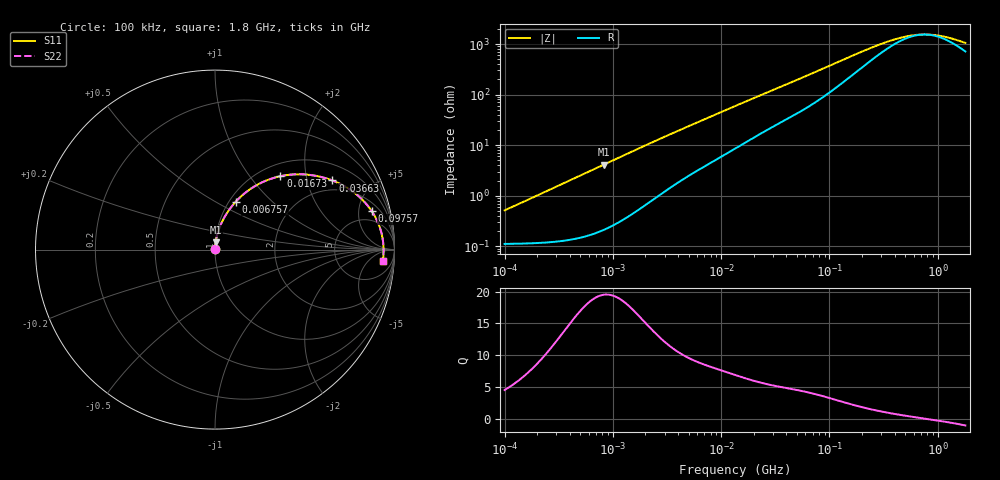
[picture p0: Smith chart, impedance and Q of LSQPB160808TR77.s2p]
! LSQPB160808TR77  S-PARAMETER MODEL  ( General Type )
! Model Generated by TAIYO YUDEN Corporation (http://www.ty-top.com)
! Version 4.0
! TAIYO YUDEN Control No. 100810NF18SB-HKC
! Copyright(c) 2007 TAIYO YUDEN CO.,LTD. All Rights Reserved.
! Product Description (link to TY-COMPAS)
! https://ds.yuden.co.jp/TYCOMPAS/or/detail?pn=LSQPB160808TR77M&u=M
! Products Name : Inductors
! Characteristics :
!  Inductance : 0.77 uH , SRF(min) : 150 MHz , DC Resistance(max) : 0.143 Ohm
!  Rated Current : Saturation :1000 mA , Temp Rise : 660 mA (40 degC)
!  Case Size : 1.6 x 0.8 / 0.063 x 0.031 [mm/inch] , Thickness : 0.8 / 0.031 [mm/inch]
!  (Conditions: Temperature = 25 degC , DC Bias Current/Voltage = 0A / 0V)
! External Node Assignments :
!  1  o---GGG---o  2
! GND o---------o GND
! Frequency Range : 0.1MHz  -  1800MHz  [ 402 STEP ]
# MHz S RI R 50
! Freq[MHz].  S11 Real  S11 Imag  S21 Real  S21 Imag  S12 Real  S12 Imag  S22 Real  S22 Imag
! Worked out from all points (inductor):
!   401 points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, 100 kHz to 1.8 GHz, reference 50 ohm
!   read as one part in series: L = 800 nH near 105 kHz
!   highest Q = 19.5 at 822 kHz (marker M1), where L = 797 nH
!   self-resonance near 751.8 MHz
!   S11 on the Smith chart (normalised r, x): 100 kHz: 1.00, +0.01; 6.757 MHz: 1.07, +0.62; 16.73 MHz: 1.23, +1.43; 36.63 MHz: 1.58, +2.87; 97.57 MHz: 3.11, +6.95; 1.8 GHz: 15, -15
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0.1  0.00114 0.00501  0.9989 -0.00501  0.9989 -0.00501  0.00114 0.00501
0.516129  0.00217 0.0258  0.9978 -0.0258  0.9978 -0.0258  0.00217 0.0258
0.822022  0.00379 0.0409  0.9962 -0.0409  0.9962 -0.0409  0.00379 0.0409
1.516485  0.00995 0.0744  0.9901 -0.0744  0.9901 -0.0744  0.00995 0.0744
2.66389  0.0262 0.1257  0.9738 -0.1257  0.9738 -0.1257  0.0262 0.1257
4.455722  0.0611 0.1947  0.9389 -0.1947  0.9389 -0.1947  0.0611 0.1947
6.757206  0.115 0.2662  0.885 -0.2662  0.885 -0.2662  0.115 0.2662
9.52142  0.1862 0.3299  0.8138 -0.3299  0.8138 -0.3299  0.1862 0.3299
13.41641  0.2866 0.3853  0.7134 -0.3853  0.7134 -0.3853  0.2866 0.3853
16.72553  0.3644 0.409  0.6356 -0.409  0.6356 -0.409  0.3644 0.409
24.15197  0.5043 0.4184  0.4957 -0.4184  0.4957 -0.4184  0.5043 0.4184
36.62703  0.6541 0.3851  0.3459 -0.3851  0.3459 -0.3851  0.6541 0.3851
50.36143  0.7492 0.3364  0.2508 -0.3364  0.2508 -0.3364  0.7492 0.3364
69.24595  0.8215 0.2774  0.1785 -0.2774  0.1785 -0.2774  0.8215 0.2774
97.57284  0.8739 0.2132  0.1261 -0.2132  0.1261 -0.2132  0.8739 0.2132
180.0045  0.9196 0.1192  0.0804 -0.1192  0.0804 -0.1192  0.9196 0.1192
357.3983  0.9355 0.0505  0.0645 -0.0505  0.0645 -0.0505  0.9355 0.0505
542.0029  0.9385 0.0208  0.0615 -0.0208  0.0615 -0.0208  0.9385 0.0208
659.3364  0.939 0.00822  0.061 -0.00822  0.061 -0.00822  0.939 0.00822
782.6622  0.9392 -0.00251  0.0608 0.00251  0.0608 0.00251  0.9392 -0.00251
1130.179  0.9386 -0.0262  0.0614 0.0262  0.0614 0.0262  0.9386 -0.0262
1800  0.9353 -0.0615  0.0647 0.0615  0.0647 0.0615  0.9353 -0.0615
